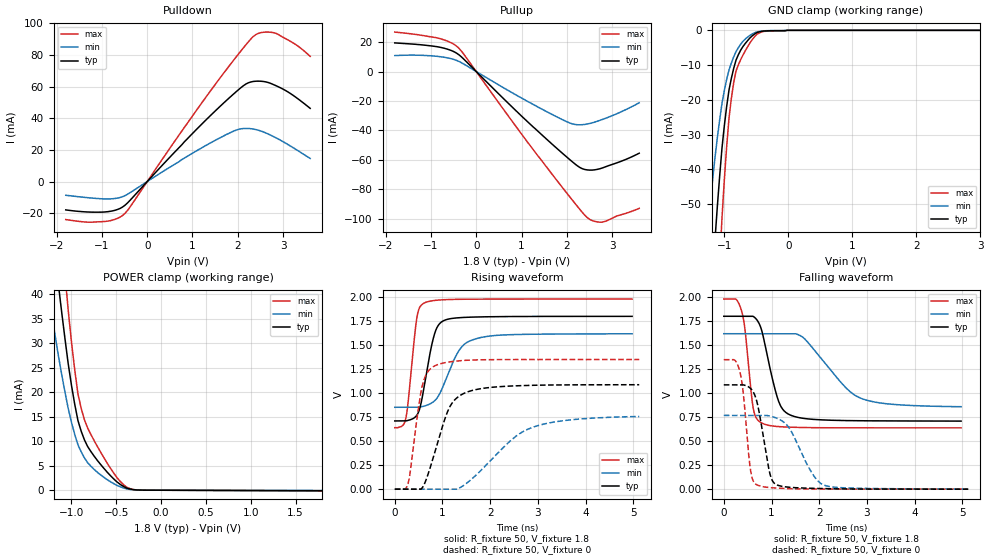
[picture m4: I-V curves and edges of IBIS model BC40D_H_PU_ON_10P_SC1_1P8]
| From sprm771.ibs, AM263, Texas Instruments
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|   Model Cell BC40D_H_PU_ON_10P_SC1_1P8
|BC40D_H_PU_ON_10P_SC1_1P8
[Model]   BC40D_H_PU_ON_10P_SC1_1P8
Model_type   I/O
Polarity   Non-Inverting
Enable   Active-Low
Vinl =  0.63
Vinh =  1.17
Cref =  15pF
Rref =  100.0000M
Vref =  0V
Vmeas =  0.9
C_comp   2.389419p   2.292106p   2.408415p
|[Input load] weak_pu_on
|[Output drive] slow
|[supplytol] 10
|[temp] ind
[Model Spec]
Vinl   0.63   0.567   0.693
Vinh   1.17   1.053   1.287
[Temperature Range]   25   125   -40
[Voltage Range]   1.8   1.62   1.98
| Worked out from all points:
|   slope of the pulldown table from 0 to 0.27 V, typ, clamps not added: 32.2 ohm
|   slope of the pullup table from 0 to 0.27 V, typ, clamps not added: 32.6 ohm
|   GND clamp passes 1 mA (typ) near -0.52 V on its own axis
|   POWER clamp passes 1 mA (typ) near -0.44 V on its own axis
|   rising waveform, R_fixture 50, V_fixture 1.8: 20-80 % time 249ps typ, 423ps min, 162ps max; typ from 0.71 V to 1.8 V
|   rising waveform, R_fixture 50, V_fixture 0: 20-80 % time 430ps typ, 996ps min, 231ps max; typ from 0 V to 1.09 V
|   falling waveform, R_fixture 50, V_fixture 1.8: 20-80 % time 310ps typ, 791ps min, 166ps max; typ from 1.8 V to 0.71 V
|   falling waveform, R_fixture 50, V_fixture 0: 20-80 % time 228ps typ, 466ps min, 151ps max; typ from 1.09 V to 0.002 V
| Nom Voltages:
|   VDD=1.1001, VDDS=1.8, VDDS18=1.8, ESD_BIASFET=0, VSS=0, VSSS=0
| Min Voltages:
|   VDD=0.99, VDDS=1.62, VDDS18=1.62, ESD_BIASFET=0, VSS=0, VSSS=0
| Max Voltages:
|   VDD=1.21, VDDS=1.98, VDDS18=1.98, ESD_BIASFET=0, VSS=0, VSSS=0
[POWER_clamp]
|   voltage   I(typ)   I(min)   I(max)
-1.8V     158.8mA    112.5mA    219.8mA
-1.255V   59.97mA    40.01mA    84.9mA
-1.145V   41.92mA    27.42mA    59.75mA
-1.109V   36.32mA    23.63mA    51.82mA
-1.073V   30.96mA    20.05mA    44.15mA
-1.036V   25.83mA    16.67mA    36.75mA
-963.6mV  17.54mA    11.39mA    24.55mA
-890.9mV  12.01mA    7.801mA    16.66mA
-818.2mV  8.875mA    5.6mA      12.63mA
-563.6mV  2.954mA    1.727mA    4.458mA
-272.7mV  55.97uA    39.41uA    57.82uA
1.8V      -99.94uA   -59.68uA   -146.8uA
[Pulldown]
|   voltage   I(typ)   I(min)   I(max)
-1.8V     -17.92mA   -8.674mA   -24.03mA
-927.3mV  -19.22mA   -10.99mA   -25.21mA
-654.5mV  -17.65mA   -10.46mA   -23.22mA
-490.9mV  -14.97mA   -8.904mA   -20.12mA
818.2mV   25.05mA    14.78mA    34.16mA
1.691V    49.7mA     28.87mA    68.59mA
2.127V    60.63mA    33.53mA    84.59mA
2.4V      63.43mA    32.84mA    92.9mA
2.618V    62.99mA    30.74mA    94.47mA
2.836V    60.69mA    27.76mA    93.76mA
3.273V    53.49mA    20.53mA    86.73mA
3.6V      46.26mA    14.64mA    79.12mA
[Pullup]
|   voltage   I(typ)   I(min)   I(max)
-1.8V     19.42mA    10.82mA    26.76mA
-818.2mV  16.58mA    10.15mA    22.47mA
-545.5mV  14.19mA    8.648mA    19.37mA
-381.8mV  11.34mA    6.842mA    15.75mA
1.036V    -31.26mA   -18.6mA    -43.9mA
1.909V    -55.59mA   -32.73mA   -78.89mA
2.182V    -62.71mA   -35.92mA   -89.46mA
2.345V    -65.94mA   -36.05mA   -95.62mA
2.455V    -66.75mA   -35.58mA   -99.18mA
2.618V    -66.67mA   -34.29mA   -101.7mA
2.782V    -65.47mA   -32.56mA   -102.2mA
3.6V      -55.4mA    -21.22mA   -92.82mA
[GND_clamp]
|   voltage   I(typ)   I(min)   I(max)
-1.8V     -270.2mA   -170.2mA   -430.1mA
-1.255V   -91.68mA   -55.92mA   -148.5mA
-1.145V   -59.94mA   -36.46mA   -97.15mA
-1.109V   -50.51mA   -30.84mA   -81.62mA
-1.073V   -41.77mA   -25.67mA   -67.14mA
-1.036V   -33.71mA   -20.94mA   -53.69mA
-927.3mV  -17.15mA   -11.38mA   -25.2mA
-854.5mV  -10.96mA   -7.657mA   -15.09mA
-781.8mV  -7.031mA   -4.995mA   -9.958mA
-563.6mV  -1.569mA   -1.036mA   -2.651mA
-18.18mV  0A         0A         0A
3.6V      0A         0A         0A
[Ramp]
| variable   typ   min   max
dV/dt_f 0.66084433/0.31279184n 0.46734565/0.81421839n 0.80984516/0.16782514n
dV/dt_r  0.6586853/0.43252091n 0.47369562/1.0506061n 0.81473948/0.23201356n
R_load = 50
[Rising Waveform]
R_fixture = 50
V_fixture = 1.8
V_fixture_min = 1.62
V_fixture_max = 1.98
|   time   V(typ)   V(min)   V(max)
0s        710.5mV    852.8mV    640.6mV
228.1ps   710.5mV    852.8mV    729.3mV
278.6ps   716.3mV    852.8mV    899.6mV
458.2ps   767.3mV    853mV      1.77V
609.1ps   1.048V     864mV      1.936V
836.3ps   1.621V     921.2mV    1.966V
1.063ns   1.763V     1.133V     1.974V
1.388ns   1.787V     1.473V     1.978V
1.775ns   1.794V     1.576V     1.979V
4.974ns   1.8V       1.618V     1.98V
[Rising Waveform]
R_fixture = 50
V_fixture = 0
V_fixture_min = 0
V_fixture_max = 0
|   time   V(typ)   V(min)   V(max)
0s        0V         0V         2.078mV
273.6ps   0V         0V         50.49mV
573.4ps   12.85mV    0V         1.07V
674.6ps   122.3mV    0V         1.209V
831.4ps   371.4mV    0V         1.283V
1.16ns    863.5mV    0V         1.327V
1.55ns    1.017V     79.03mV    1.344V
2.456ns   1.074V     517.5mV    1.35V
2.875ns   1.082V     641.7mV    1.35V
5.123ns   1.088V     756.5mV    1.35V
[Falling Waveform]
R_fixture = 50
V_fixture = 1.8
V_fixture_min = 1.62
V_fixture_max = 1.98
|   time   V(typ)   V(min)   V(max)
0s        1.801V     1.619V     1.98V
369ps     1.801V     1.619V     1.862V
442ps     1.801V     1.619V     1.673V
618.1ps   1.799V     1.619V     841.6mV
787.4ps   1.665V     1.619V     692.4mV
1.129ns   945.2mV    1.619V     653.9mV
1.381ns   776.1mV    1.619V     647mV
1.677ns   738mV      1.574V     643.2mV
2.853ns   713.9mV    952.2mV    639.9mV
4.974ns   710.2mV    859.9mV    639.7mV
[Falling Waveform]
R_fixture = 50
V_fixture = 0
V_fixture_min = 0
V_fixture_max = 0
|   time   V(typ)   V(min)   V(max)
0s        1.087V     769.5mV    1.349V
333.6ps   1.087V     769.5mV    1.23V
404.9ps   1.087V     769.5mV    1.017V
557ps     1.052V     769.5mV    210.7mV
685.7ps   927.1mV    769.5mV    49.13mV
959.4ps   177.6mV    763.4mV    18.56mV
1.117ns   45.79mV    739mV      13.61mV
1.37ns    22.17mV    640mV      7.167mV
2.109ns   7.6mV      42.83mV    3.034mV
5.123ns   2.08mV     3.321mV    2.564mV
